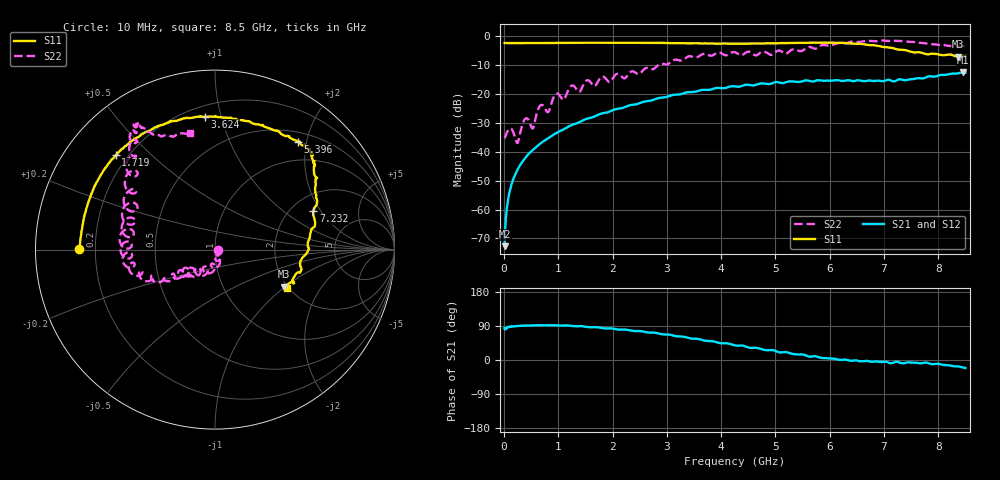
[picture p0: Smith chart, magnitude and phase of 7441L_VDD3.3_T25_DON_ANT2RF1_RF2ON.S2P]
!Agilent Technologies,E5071C,MY46417908,A.11.23
!Date: Mon May 03 19:53:55 2021
!Data & Calibration Information:
!Freq	S11:SOLT2(ON)	S21:SOLT2(ON)	S12:SOLT2(ON)	S22:SOLT2(ON)
!PortZ  Port1:50+j0  Port2:50+j0
!Above PortZ is port z conversion or system Z0 setting when saving the data.
!When reading, reference impedance value at option line is always used.
# Hz S dB R 50
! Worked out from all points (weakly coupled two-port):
!   1601 points, 10 MHz to 8.5 GHz, reference 50 ohm
!   highest |S21| = -12.62 dB at 8.458 GHz (marker M1); lowest = -72.7 dB at 10 MHz (marker M2)
!   lowest |S11| = -7.2 dB at 8.357 GHz (marker M3), VSWR 2.56, Z = 96.3 - j49.3 ohm
!   |S11| at or under -10 dB: nowhere
!   |S22| runs from -37.0 to -1.6 dB; largest |S21 - S12| = 0.0051
!   S11 on the Smith chart (normalised r, x): 10 MHz: 0.14, +0.00; 1.719 GHz: 0.16, +0.39; 3.624 GHz: 0.27, +0.89; 5.396 GHz: 0.65, +1.85; 7.232 GHz: 2.61, +1.71; 8.5 GHz: 1.96, -1.04
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1e7  -2.42 179.6  -72.65 83.8  -72.33 83.6  -35.30 1.1
6.836875e7  -2.47 178.0  -57.37 85.8  -57.26 86.5  -32.72 -7.5
1.214312e8  -2.47 176.4  -52.32 88.3  -52.35 88.0  -31.99 -28.2
2.43475e8  -2.49 172.9  -46.36 89.6  -46.35 89.7  -37.00 -36.1
3.336812e8  -2.49 170.4  -43.58 90.5  -43.56 90.5  -30.86 -28.4
4.13275e8  -2.50 168.1  -41.66 90.9  -41.65 91.0  -28.44 -59.2
5.300125e8  -2.48 165.1  -39.40 90.9  -39.40 91.0  -31.98 -59.4
6.573625e8  -2.47 161.7  -37.36 91.8  -37.36 91.8  -24.30 -62.7
8.112438e8  -2.45 157.8  -35.36 91.8  -35.39 91.8  -26.33 -78.2
9.598188e8  -2.41 153.8  -33.56 91.5  -33.57 91.5  -19.98 -87.4
1.426769e9  -2.37 143.1  -29.44 89.4  -29.44 89.3  -18.29 -109.0
1.718612e9  -2.35 136.5  -27.36 86.4  -27.36 86.4  -16.12 -121.8
2.843538e9  -2.46 111.7  -21.49 70.0  -21.50 70.1  -10.02 -145.9
3.623556e9  -2.59 94.5  -18.72 54.1  -18.74 53.9  -6.62 -161.9
4.255e9  -2.65 77.6  -17.44 38.4  -17.43 37.9  -5.66 177.8
5.395844e9  -2.41 52.5  -15.84 14.5  -15.80 14.1  -4.92 143.6
5.671769e9  -2.30 49.1  -15.76 9.2  -15.72 8.7  -4.02 135.6
7.088538e9  -3.96 26.5  -15.16 -7.3  -15.18 -7.8  -1.75 122.4
7.231806e9  -4.61 21.4  -15.39 -4.5  -15.36 -5.1  -1.71 121.3
8.356731e9  -7.17 -28.2  -12.95 -16.9  -12.99 -17.0  -3.41 106.1
8.45755e9  -6.95 -27.6  -12.62 -19.9  -12.66 -19.7  -3.57 103.3
8.5e9  -6.89 -27.9  -12.68 -21.1  -12.71 -21.0  -3.54 102.2
